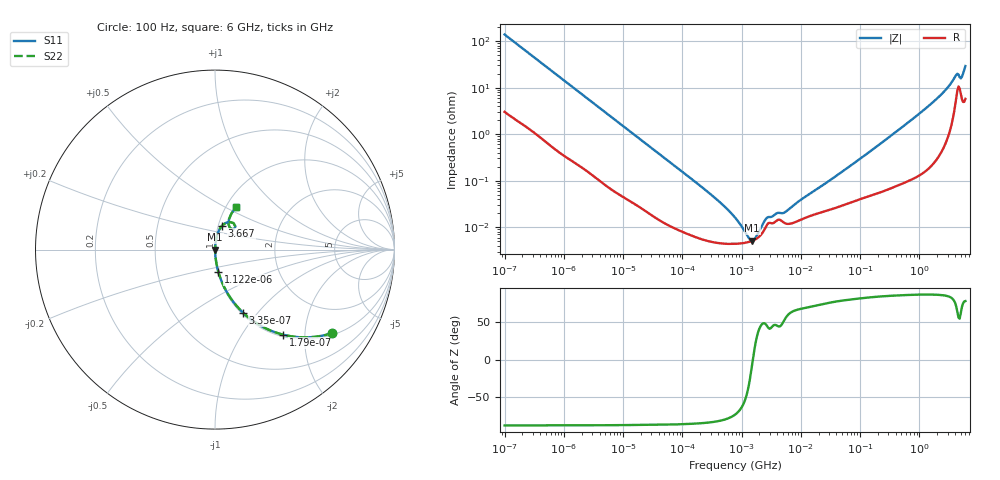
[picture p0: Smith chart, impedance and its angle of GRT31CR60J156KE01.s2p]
!Murata Part Number: GRT31CR60J156KE01
!These Parameters are Measured in Series Mode Connection
!Data Generated on Jun 19, 2026
!  o--ll--o
!Port1  Port2
!  o------o
!Operation Temp=25[degC], DC Bias Voltage=0[V]
!Freq. Start=100[Hz] Stop=6[GHz] 401[Steps]
# Hz S RI R 50
!Freq.(Hz) S11(Real) S11(Imag) S21(Real) S21(Imag) S12(Real) S12(Imag) S22(Real) S22(Imag)
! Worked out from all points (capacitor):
!   401 points, 100 Hz to 6 GHz, reference 50 ohm
!   read as one part in series: C = 11.4 uF near 109 Hz
!   lowest |Z| = 5.12 mohm at 1.516 MHz (marker M1)
!   series resonance near 1.552 MHz, so ESL is about 920 pH
!   S11 on the Smith chart (normalised r, x): 100 Hz: 1.06, -2.77; 179 Hz: 1.04, -1.56; 335 Hz: 1.02, -0.84; 1.122 kHz: 1.01, -0.26; 3.667 GHz: 1.04, +0.28; 6 GHz: 1.11, +0.57
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100  0.6546 -0.4648  0.3454 0.4648  0.3454 0.4648  0.6546 -0.4648
179  0.3813 -0.4744  0.6187 0.4744  0.6187 0.4744  0.3813 -0.4744
335  0.1567 -0.3517  0.8433 0.3517  0.8433 0.3517  0.1567 -0.3517
573  0.0629 -0.2313  0.9371 0.2313  0.9371 0.2313  0.0629 -0.2313
1122  0.0191 -0.1251  0.9809 0.1251  0.9809 0.1251  0.0191 -0.1251
2008  0.00706 -0.0715  0.9929 0.0715  0.9929 0.0715  0.00706 -0.0715
40335  0.000157 -0.00379  0.9998 0.00379  0.9998 0.00379  0.000157 -0.00379
316350  4.82e-05 -0.00048  1 0.00048  1 0.00048  4.82e-05 -0.00048
774597  4.38e-05 -0.000156  1 0.000156  1 0.000156  4.38e-05 -0.000156
1059725  4.54e-05 -8.15e-05  1 8.15e-05  1 8.15e-05  4.54e-05 -8.15e-05
1516199  5.1e-05 -5e-06  0.9999 5e-06  0.9999 5e-06  5.1e-05 -5e-06
2074311  6.62e-05 6.48e-05  0.9999 -6.48e-05  0.9999 -6.48e-05  6.62e-05 6.48e-05
2713602  0.000115 0.000113  0.9999 -0.000113  0.9999 -0.000113  0.000115 0.000113
4060267  0.000143 0.000143  0.9999 -0.000143  0.9999 -0.000143  0.000143 0.000143
5311619  0.000123 0.000167  0.9999 -0.000167  0.9999 -0.000167  0.000123 0.000167
1.555665e7  0.000181 0.000535  0.9998 -0.000535  0.9998 -0.000535  0.000181 0.000535
3.124326e8  0.000737 0.00867  0.9993 -0.00867  0.9993 -0.00867  0.000737 0.00867
1.712697e9  0.00465 0.0485  0.9954 -0.0485  0.9954 -0.0485  0.00465 0.0485
3.666503e9  0.0384 0.1314  0.9616 -0.1314  0.9616 -0.1314  0.0384 0.1314
4.193612e9  0.0813 0.154  0.9187 -0.154  0.9187 -0.154  0.0813 0.154
5.016141e9  0.0835 0.1193  0.9165 -0.1193  0.9165 -0.1193  0.0835 0.1193
6e9  0.1183 0.2379  0.8817 -0.2379  0.8817 -0.2379  0.1183 0.2379
